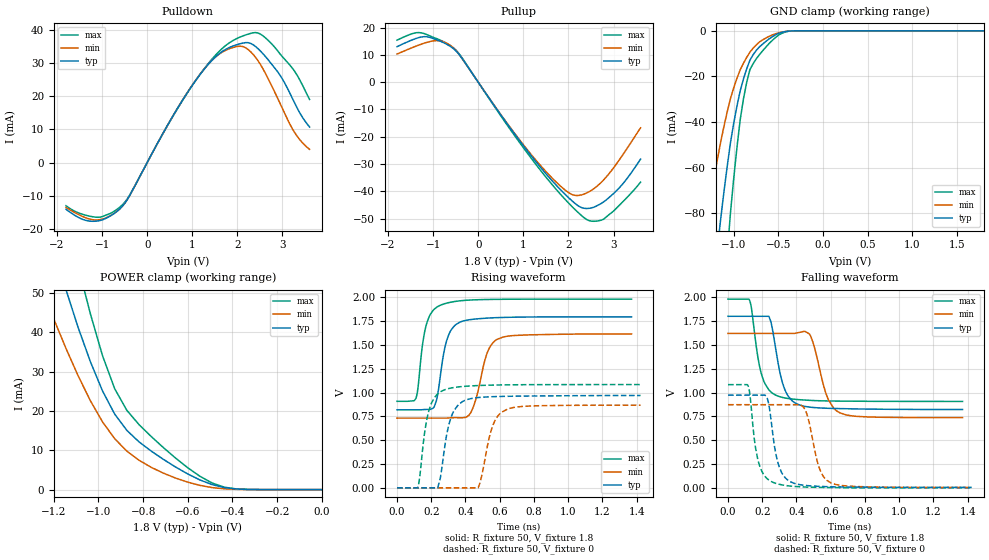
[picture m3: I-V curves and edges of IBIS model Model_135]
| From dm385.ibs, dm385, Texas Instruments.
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| Model based on original model for BCSHTLTCSCDVPBFZ_SSDHV
|   Sub model SR00_9MA_10PER_1P8
[model]   Model_135
|[Description]  [1.8V-3-STATE-NOTERM-FASTEST:9MA, IND, 10%]
|   Fastest slew rate (SR[1:0] = "00"), 0.88 * RExt = 1.125 * Iout
|   (I[2:0] = "100"), 9mA nominal with Rext = 50R,ODT off (ODT[1:0]
|   = "00") CMOS mode,Industrial temperature range (-40C to 125C,
|   25C nominal),10% power supply tolerance
|[Input Load]   NOTERM
|[Output Drive] FASTEST:9MA
|Voltage   1.8V
|Mode   3-STATE
Model_type   3-state
Polarity   Non-Inverting
Enable   Active-Low
Cref =  15pF
Rref =  100.0000M
Vref =  0V
Vmeas =  0.9
C_comp   1.851324p   1.663768p   1.973575p
[Temperature Range]   25   125   -40
[Voltage Range]   1.8   1.62   1.98
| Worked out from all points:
|   slope of the pulldown table from 0 to 0.27 V, typ, clamps not added: 39.3 ohm
|   slope of the pullup table from 0 to 0.27 V, typ, clamps not added: 41.3 ohm
|   GND clamp passes 1 mA (typ) near -0.49 V on its own axis
|   POWER clamp passes 1 mA (typ) near -0.47 V on its own axis
|   rising waveform, R_fixture 50, V_fixture 1.8: 20-80 % time 60ps typ, 75.2ps min, 54.5ps max; typ from 0.819 V to 1.79 V
|   rising waveform, R_fixture 50, V_fixture 0: 20-80 % time 62.8ps typ, 68.9ps min, 57.6ps max; typ from 0 V to 0.969 V
|   falling waveform, R_fixture 50, V_fixture 1.8: 20-80 % time 69.9ps typ, 80.8ps min, 63.3ps max; typ from 1.8 V to 0.822 V
|   falling waveform, R_fixture 50, V_fixture 0: 20-80 % time 57.8ps typ, 67.9ps min, 53ps max; typ from 0.973 V to 0.005 V
[POWER_clamp]
-1.8V     194.9mA    137.1mA    262.8mA
-1.236V   68.49mA    48.51mA    92.67mA
-1.145V   50.76mA    35.86mA    69.65mA
-1.127V   47.56mA    33.54mA    65.34mA
-1.055V   35.4mA     24.69mA    48.69mA
-981.8mV  25.06mA    17.2mA     34.01mA
-927.3mV  19.17mA    12.93mA    25.61mA
-872.7mV  15.03mA    9.767mA    20.12mA
-818.2mV  12.12mA    7.45mA     16.5mA
-654.5mV  5.738mA    2.93mA     8.003mA
-436.4mV  508.2uA    199.4uA    613uA
0V        2.273nA    15.95nA    16.67nA
[Pulldown]
-1.8V     -14.14mA   -13.59mA   -13.06mA
-1.145V   -17.74mA   -17.37mA   -16.51mA
-545.5mV  -13.15mA   -13.12mA   -12.71mA
545.5mV   13.5mA     13.52mA    13.41mA
1.091V    25.12mA    25.21mA    25.13mA
1.527V    32.11mA    32.07mA    32.67mA
1.964V    35.54mA    35.01mA    37.35mA
2.291V    36.06mA    33.55mA    39.05mA
2.618V    32.13mA    27.06mA    37.75mA
2.945V    26.42mA    17.9mA     32.85mA
3.218V    19.44mA    10.24mA    28.56mA
3.6V      10.76mA    3.999mA    19.09mA
[Pullup]
-1.8V     12.99mA    10.3mA     15.38mA
-1.2V     16.67mA    14.26mA    17.79mA
-872.7mV  15.21mA    15.17mA    15.62mA
-600mV    12.91mA    13.24mA    13.19mA
-381.8mV  9.242mA    9.222mA    9.473mA
1.2V      -27.49mA   -27.01mA   -28.42mA
1.745V    -38.03mA   -36.86mA   -39.59mA
2.127V    -44.16mA   -41.42mA   -46.35mA
2.455V    -46.24mA   -40.18mA   -50.71mA
2.727V    -44.44mA   -36.72mA   -50.57mA
3.164V    -38.07mA   -27.64mA   -44.53mA
3.6V      -28.19mA   -16.75mA   -36.64mA
[GND_clamp]
-1.8V     -346.1mA   -209.3mA   -568.3mA
-1.327V   -149.7mA   -89.03mA   -250.9mA
-1.291V   -135.6mA   -80.47mA   -227.5mA
-1.145V   -82.35mA   -48.67mA   -137.7mA
-1.073V   -59.44mA   -35.55mA   -97.96mA
-1.036V   -49.1mA    -29.72mA   -79.9mA
-927.3mV  -26.31mA   -17.11mA   -38.99mA
-854.5mV  -16.67mA   -11.64mA   -22.56mA
-818.2mV  -12.86mA   -9.351mA   -16.98mA
-672.7mV  -5.705mA   -3.913mA   -8.624mA
-381.8mV  -120.4uA   -129uA     -167.4uA
1.8V      2.273nA    454nA      6.646nA
[Ramp]
dV/dt_f 0.59844723/70.630322p  0.5448731/81.605134p 0.65033969/63.406141p
dV/dt_r 0.59103683/63.385422p 0.53601986/70.026212p 0.65645762/57.630194p
R_load = 50
[Rising Waveform]
R_fixture = 50
V_fixture = 1.8
V_fixture_min = 1.62
V_fixture_max = 1.98
0s        818.8mV    731.7mV    908mV
110.8ps   818.8mV    731.7mV    938.9mV
169.7ps   822.6mV    731.7mV    1.701V
217.6ps   851.4mV    731.7mV    1.874V
255.7ps   1.209V     731.7mV    1.918V
311.6ps   1.642V     734.5mV    1.947V
421.4ps   1.763V     764.2mV    1.97V
529.1ps   1.781V     1.426V     1.976V
584ps     1.786V     1.557V     1.978V
1.37ns    1.794V     1.615V     1.98V
[Rising Waveform]
R_fixture = 50
V_fixture = 0
V_fixture_min = 0
V_fixture_max = 0
0s        0V         0V         0V
119.8ps   0V         0V         0V
185.7ps   0V         0V         806.3mV
237.9ps   0V         0V         985.8mV
273.3ps   361.1mV    0V         1.025V
332.6ps   809.2mV    0V         1.053V
473.1ps   947.2mV    0V         1.073V
555.8ps   956.3mV    634.5mV    1.078V
646.8ps   960.5mV    827.6mV    1.081V
1.423ns   969mV      867.5mV    1.084V
[Falling Waveform]
R_fixture = 50
V_fixture = 1.8
V_fixture_min = 1.62
V_fixture_max = 1.98
0s        1.801V     1.621V     1.981V
126.6ps   1.801V     1.621V     1.966V
197.1ps   1.801V     1.621V     1.184V
238.6ps   1.801V     1.621V     1.029V
285.1ps   1.389V     1.621V     968.3mV
350.7ps   964.9mV    1.621V     938mV
475.9ps   847.8mV    1.615V     918.6mV
585.8ps   835.1mV    926.1mV    912.1mV
655.4ps   831.9mV    786.1mV    910.5mV
1.37ns    822mV      737mV      907.1mV
[Falling Waveform]
R_fixture = 50
V_fixture = 0
V_fixture_min = 0
V_fixture_max = 0
0s        972.9mV    872.9mV    1.083V
118.1ps   972.9mV    872.9mV    1.068V
173.6ps   972.9mV    872.9mV    301.5mV
230.9ps   931.2mV    872.9mV    92.81mV
261.2ps   569.9mV    872.9mV    59.37mV
315.4ps   153.2mV    872.9mV    31.33mV
440.6ps   27.88mV    848.3mV    9.646mV
532.3ps   15.8mV     213.7mV    5.12mV
601.7ps   11.48mV    51.71mV    3.37mV
1.423ns   4.777mV    4.648mV    0V
